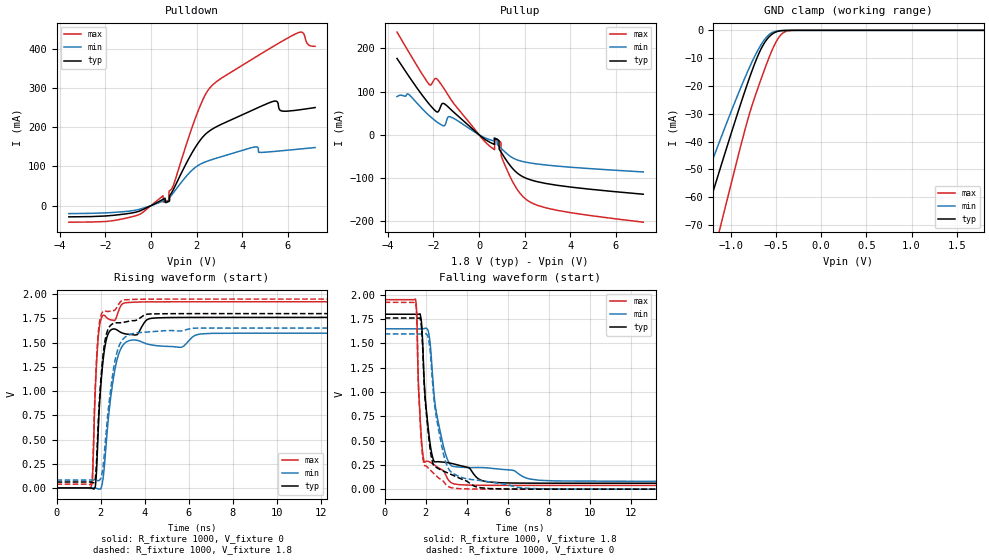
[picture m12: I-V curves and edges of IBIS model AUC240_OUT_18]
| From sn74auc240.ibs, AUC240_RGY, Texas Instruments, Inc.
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[Model]   AUC240_OUT_18
Model_type  3-state
Enable   Active-Low
Vref =   0
Rref =   1000
Cref =   30p
Vmeas =   0.9
| variable   typ   min   max
C_comp   5.63pF   5.09pF   5.91pF
| C_pullup   6.43pF   0.72pF   12.09pF
| C_pulldown   6.34pF   3.26pF   13.65pF
| C_tri-state   5.63pF   5.09pF   5.91pF
[Temperature Range]   40   100   -40
| Ambient temperature   25   85   -40
[Voltage range]   1.8   1.65   1.95
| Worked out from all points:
|   slope of the pulldown table from 0 to 0.27 V, typ, clamps not added: 34.2 ohm
|   slope of the pullup table from 0 to 0.27 V, typ, clamps not added: 24.6 ohm
|   GND clamp passes 1 mA (typ) near -0.53 V on its own axis
|   rising waveform, R_fixture 1000, V_fixture 0: 20-80 % time 314ps typ, 494ps min, 213ps max; typ from 0 V to 1.76 V
|   falling waveform, R_fixture 1000, V_fixture 1.8: 20-80 % time 394ps typ, 643ps min, 237ps max; typ from 1.8 V to 0.061 V
|   rising waveform, R_fixture 1000, V_fixture 1.8: 20-80 % time 313ps typ, 490ps min, 211ps max; typ from 0.061 V to 1.8 V
|   falling waveform, R_fixture 1000, V_fixture 0: 20-80 % time 396ps typ, 645ps min, 237ps max; typ from 1.76 V to 0 V
[GND Clamp]
| AUC240_OUT_18
|   Voltage   I(typ)   I(min)   I(max)
-3.6V     -319.1mA   -267.5mA   -389.1mA
-1.48V    -88.18mA   -70.9mA    -117.8mA
-1.435V   -83.33mA   -66.9mA    -111.9mA
-1.3V     -68.86mA   -54.99mA   -94.42mA
-1.105V   -48.23mA   -38.17mA   -69.07mA
-830mV    -20.41mA   -15.93mA   -34.03mA
-685mV    -7.947mA   -6.184mA   -19.28mA
-565mV    -1.95mA    -1.227mA   -8.764mA
-490mV    -463.9uA   -241.5uA   -3.576mA
-425mV    -91.37uA   -53.53uA   -985.3uA
-300mV    -2.288uA   -2.898uA   -16.98uA
1.8V      674.8pA    50.15nA    728.7pA
[Pulldown]
| AUC240_OUT_18
|   Voltage   I(typ)   I(min)   I(max)
-3.6V     -28.49mA   -20.22mA   -42.08mA
-1.155V   -21.32mA   -15.05mA   -32.66mA
530mV     16.28mA    11.83mA    25.26mA
780mV     11.04mA    10.74mA    14.1mA
800mV     11.66mA    11.63mA    36.72mA
1.97V     150.9mA    98.78mA    226.4mA
2.645V    193.6mA    117.1mA    304.4mA
4.56V     246.4mA    149.8mA    377.8mA
5.38V     266.3mA    138.2mA    406.7mA
5.71V     242mA      140mA      417.9mA
6.445V    244mA      144mA      440.9mA
7.2V      250.3mA    148.3mA    406.4mA
[Pullup]
| AUC240_OUT_18
|   Voltage   I(typ)   I(min)   I(max)
-3.6V     176.5mA    88.25mA    237.5mA
-2.185V   70.84mA    44.34mA    116.3mA
-1.835V   52.55mA    29.22mA    128.3mA
-1.53V    71.89mA    20.76mA    106.1mA
-1.26V    59.61mA    41.57mA    83.77mA
480mV     -17.54mA   -11.58mA   -26.82mA
845mV     -12.04mA   -24.63mA   -13.29mA
940mV     -38.16mA   -29.53mA   -16.81mA
980mV     -41.36mA   -31.67mA   -49.57mA
1.26V     -63.84mA   -45.45mA   -85.39mA
2.065V    -100.5mA   -63.4mA    -149.4mA
7.2V      -137.3mA   -85.82mA   -202mA
[Ramp]
| AUC240_OUT_18
| variable   typ   min   max
dV/dt_r   1.06/3.15E-10   0.97/5.00E-10   1.16/2.14E-10
dV/dt_f   1.05/3.95E-10   0.95/6.50E-10   1.15/2.39E-10
R_load = 1000
[Rising Waveform]
| AUC240_OUT_18
R_fixture =   1000
C_fixture =   0
L_fixture =   0
V_fixture =   0
V_fixture_min = 0
V_fixture_max = 0
|   Time   V(typ)   V(min)   V(max)
0s        10.65nV    37.28nV    1.248nV
1.605ns   -3.699mV   1.101mV    37.53mV
1.785ns   67.8mV     -2.352mV   1.136V
1.895ns   603.1mV    -10.52mV   1.554V
2.015ns   1.069V     -7.622mV   1.741V
2.35ns    1.594V     709.3mV    1.745V
2.69ns    1.637V     1.268V     1.745V
3.08ns    1.593V     1.491V     1.91V
4.9ns     1.758V     1.463V     1.922V
34.99ns   1.761V     1.597V     1.922V
[Falling Waveform]
| AUC240_OUT_18
R_fixture =   1000
C_fixture =   0
L_fixture =   0
V_fixture =   1.8
V_fixture_min = 1.65
V_fixture_max = 1.95
|   Time   V(typ)   V(min)   V(max)
0s        1.8V       1.65V      1.95V
1.5ns     1.799V     1.65V      1.952V
1.65ns    1.8V       1.649V     1.052V
1.8ns     1.697V     1.649V     486.5mV
1.95ns    1.017V     1.654V     276.2mV
2.11ns    650.6mV    1.636V     286.6mV
2.555ns   282.8mV    746.9mV    229.3mV
3.395ns   258.3mV    232.5mV    53.47mV
5.725ns   65.22mV    203.3mV    39.07mV
34.99ns   61.08mV    81.02mV    38.7mV
[Rising Waveform]
| AUC240_OUT_18
R_fixture =   1000
C_fixture =   0
L_fixture =   0
V_fixture =   1.8
V_fixture_min = 1.65
V_fixture_max = 1.95
|   Time   V(typ)   V(min)   V(max)
0s        61.05mV    81.01mV    38.68mV
1.56ns    60.27mV    81.84mV    47.83mV
1.63ns    56.31mV    81.98mV    131.7mV
1.77ns    115.9mV    79.76mV    1.102V
1.965ns   968.6mV    83.71mV    1.729V
2.11ns    1.366V     218.8mV    1.822V
2.29ns    1.608V     668.8mV    1.822V
2.645ns   1.703V     1.302V     1.835V
3.025ns   1.709V     1.539V     1.94V
34.99ns   1.8V       1.65V      1.95V
[Falling Waveform]
| AUC240_OUT_18
R_fixture =   1000
C_fixture =   0
L_fixture =   0
V_fixture =   0
V_fixture_min = 0
V_fixture_max = 0
|   Time   V(typ)   V(min)   V(max)
0s        1.761V     1.597V     1.922V
1.5ns     1.76V      1.597V     1.923V
1.65ns    1.76V      1.597V     1.032V
1.795ns   1.661V     1.596V     462mV
1.95ns    983.9mV    1.599V     242.1mV
2.1ns     626.1mV    1.575V     223.6mV
2.515ns   223.9mV    742mV      135.7mV
3.235ns   152.1mV    177.1mV    15.71mV
7.435ns   574.4uV    4.565mV    154.6uV
34.99ns   35.51uV    3.065uV    15.46uV
